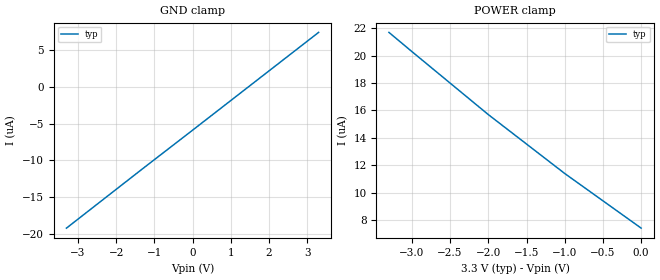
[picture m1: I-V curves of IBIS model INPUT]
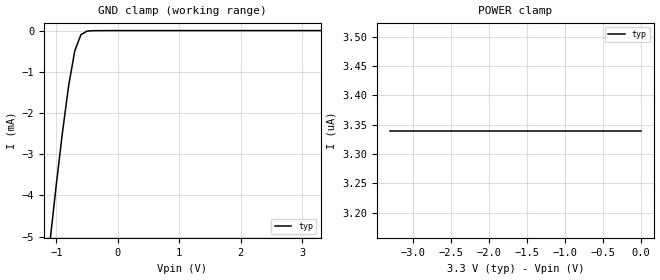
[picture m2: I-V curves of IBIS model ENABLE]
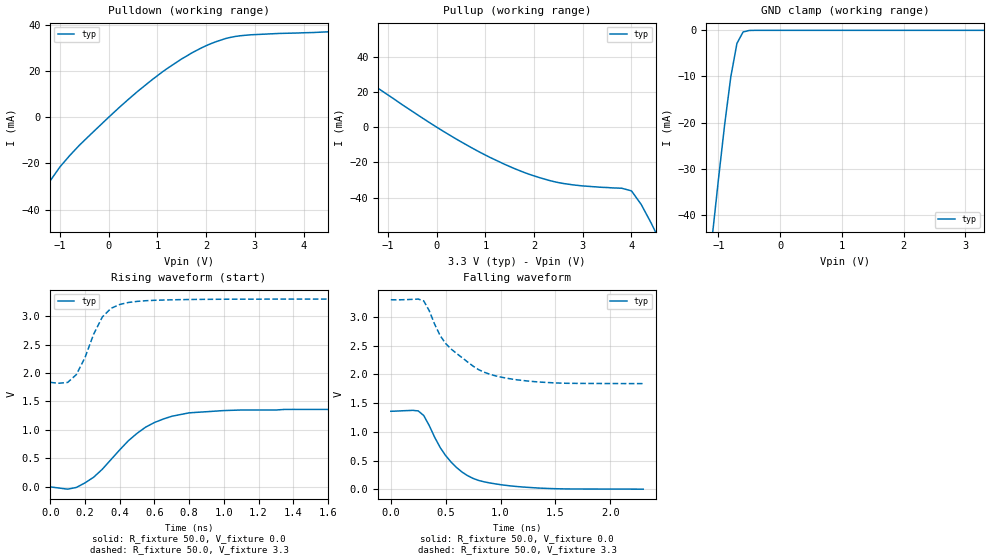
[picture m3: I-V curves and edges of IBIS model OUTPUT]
|   Texas Instruments Incorporated
|   Data Transmissions Products
|   IBIS Model for SN55LVDS33
|   16W CPK Package
[IBIS Ver]   3.2
[Comment char]   |_char
[File name]   lvds33w.ibs
[File Rev]   1.0
[Date]   26Mar01
[Source]   File originated at Texas Instruments Incorporated.
   Data Transmission Products Group. All data based on
   Bench Measurements.
[Notes]
   This file was modified on 4/14/2014 14:11 by the Mentor Graphics
   IBISVTC program, to remove initial non-switching delay(s) from one
   or more models V-t tables. Modified models:
   OUTPUT
   Original V-t tables have been left in the affected models, but commented out.
[Disclaimer]
(C) Copyright Texas Instruments Incorporated 2001
   All rights reserved
  Texas Instruments Incorporated hereby grants the user of this IBIS
model a non-exclusive, nontransferable license to use this IBIS model
under the following terms.  Before using this IBIS model, the user
should read this license.  If the user does not accept these terms,
the IBIS model should be returned to Texas Instruments within 30 days.
  The user is granted this license only to use the IBIS model and
is not granted rights to sell, load, rent, lease or license the IBIS
model in whole or in part, or in modified form to anyone other than
user.  User may modify the IBIS model to suit its specific applications
but rights to derivative works and such modifications shall belong to
Texas Instruments.
  This IBIS model is provided on an "AS IS" basis and Texas Instruments
makes absolutely no warranty with respect to the information contained
herein.  TEXAS INSTRUMENTS DISCLAIMS AND CUSTOMER WAIVES ALL WARRANTIES,
EXPRESS OR IMPLIED, INCLUDING WARRANTIES OF MERCHANTABILITY OR FITNESS
FOR A PARTICULAR PURPOSE. The entire risk as to quality and performance
is with the Customer. ACCORDINGLY, IN NO EVENT SHALL THE COMPANY BE LIABLE
FOR ANY DAMAGES, WHETHER IN CONTRACT OR TORT,INCLUDING ANY LOST PROFITS
OR OTHER INCIDENTAL, CONSEQUENTIAL, EXEMPLARY, OR PUNITIVE DAMAGES ARISING
OUT OF THE USE OR APPLICATION OF THE IBIS model provided in this package.
Further, Texas Instruments reserves the right to discontinue or make changes
without notice to any product herein to improve reliability, function, or
design. Texas Instruments does not convey any license under patent rights
or any other intellectual property rights, including those of third parties.
Contact Texas Instruments at ATTN:DATA TRANSMISSIONS
[Copyright]   Copyright 2001, Texas Instruments, All Rights Reserved
[Component]   SN55LVDS33W
[Manufacturer]  Texas Instruments Incorporated
[Package]
|   typ   min   max
R_pkg   0.177   0.141   0.245
L_pkg   3.23e-9   2.617e-9   4.412e-9
C_pkg   1.228e-12   1.057e-12   1.531e-12
[Pin]   signal_name   model_name   R_pin   L_pin   C_pin
1   1B   INPUT   0.244   4.385e-9 1.524e-12
2   1A   INPUT   0.176   3.183e-9 1.235e-12
3   1Y   OUTPUT   0.142   2.637e-9 1.071e-12
4   G   ENABLE   0.144   2.645e-9 1.060e-12
5   2Y   OUTPUT   0.147   2.708e-9 1.081e-12
6   2A   INPUT   0.144   2.687e-9 1.092e-12
7   2B   INPUT   0.176   3.182e-9 1.236e-12
8   GND   GND   0.245   4.412e-9 1.531e-12
9   3B   INPUT   0.245   4.411e-9 1.531e-12
10   3A   INPUT   0.176   3.183e-9 1.235e-12
11   3Y   OUTPUT   0.141   2.617e-9 1.063e-12
12   /G   ENABLE   0.144   2.639e-9 1.057e-12
13   4Y   OUTPUT   0.150   2.772e-9 1.102e-12
14   4A   INPUT   0.141   2.617e-9 1.063e-12
15   4B   INPUT   0.176   3.182e-9 1.235e-12
16   VCC   POWER   0.245   4.411e-9 1.531e-12
[Diff_pin]   inv_pin   vdiff   tdelay_typ   tdelay_min   tdelay_max
| The 'xA' pin is Diff_pin and the 'xB' pin is the inv_pin
2   1   50mV   0 0 0   | Vth  +/-50mV
6   7   50mV   0 0 0
10   9   50mV   0 0 0
14   15   50mV   0 0 0
| Models and submodels in the file (3): INPUT (Input), ENABLE (Input), OUTPUT (3-state)
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|   Receiver Input  MODEL
[Model]   INPUT
Model_type   Input
|Signals   1A,1B,2A,2B,3A,3B,4A,4B
Vinh = 2.0
Vinl = 0.8
|   typ   min   max
C_comp   1.0pF   NA   NA
|   typ   min   max
[Temperature Range]   25.0   NA   NA
[Voltage range]   3.3V   3.0V   3.6V
[GND_clamp]
|   Voltage   I(typ)   I(min)   I(max)
-3.3V     -19.2uA    NA         NA
-1.3V     -11.1uA    NA         NA
0V        -5.89uA    NA         NA
1.3V      -651nA     NA         NA
3.3V      7.41uA     NA         NA
[Power_clamp]
| Note that the[POWER_clamp]voltage table is referenced to Vcc
| and is calculated using Vtable=Vcc - Vmeasured.
|   Voltage   I(typ)   I(min)   I(max)
-3.3V     21.7uA     NA         NA
-3V       20.3uA     NA         NA
-2V       15.7uA     NA         NA
-1V       11.4uA     NA         NA
0V        7.41uA     NA         NA
|   Receiver Enable  MODEL
[Model]   ENABLE
Model_type   Input
|Signals   G,/G
Vinh = 2.0
Vinl = 0.8
|   typ   min   max
C_comp   1.0pF   NA   NA
|   typ   min   max
[Temperature Range]   25.0   NA   NA
[Voltage range]   3.3V   3.0V   3.6V
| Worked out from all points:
|   GND clamp passes 1 mA (typ) near -0.76 V on its own axis
[GND_clamp]
|   Voltage   I(typ)   I(min)   I(max)
-3.3V     -43.1mA    NA         NA
-1.1V     -5.08mA    NA         NA
-1V       -3.73mA    NA         NA
-900mV    -2.47mA    NA         NA
-800mV    -1.34mA    NA         NA
-700mV    -493uA     NA         NA
-600mV    -98.5uA    NA         NA
-500mV    -13.3uA    NA         NA
3.3V      3.34pA     NA         NA
[Power_clamp]
| Note that the[POWER_clamp]voltage table is referenced to Vcc
| and is calculated using Vtable=Vcc - Vmeasured.
|   Voltage   I(typ)   I(min)   I(max)
-3.3V     3.34uA     NA         NA
-2.7V     3.34uA     NA         NA
-2V       3.34uA     NA         NA
-800mV    3.34uA     NA         NA
0V        3.34uA     NA         NA
|   Receiver Output  MODEL
[Model]   OUTPUT
Model_type   3-state
| Signals   1Y,2Y,3Y,4Y
Vmeas = 1.5V   |Reference voltage for timing measurements
Cref = 8pF   |Timing specification test load capacitance value
Vref = 0   |Timing specification test load voltage; GND
| variable   typ   min   max
C_comp   1.0pF   NA   NA
|   typ   min   max
[Temperature Range]   25.0   NA   NA
[Voltage range]   3.3V   3.0V   3.6V
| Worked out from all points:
|   slope of the pulldown table from 0 to 0.495 V, typ, clamps not added: 52.7 ohm
|   slope of the pullup table from 0 to 0.495 V, typ, clamps not added: 60.3 ohm
|   GND clamp passes 1 mA (typ) near -0.63 V on its own axis
|   rising waveform, R_fixture 50.0, V_fixture 0.0: 20-80 % time 287ps typ, NA min, NA max; typ from 0 V to 1.36 V
|   falling waveform, R_fixture 50.0, V_fixture 0.0: 20-80 % time 315ps typ, NA min, NA max; typ from 1.36 V to 0.004 V
|   rising waveform, R_fixture 50.0, V_fixture 3.3: 20-80 % time 131ps typ, NA min, NA max; typ from 1.84 V to 3.3 V
|   falling waveform, R_fixture 50.0, V_fixture 3.3: 20-80 % time 389ps typ, NA min, NA max; typ from 3.3 V to 1.84 V
[Pulldown]
|   Voltage   I(typ)   I(min)   I(max)
-3.3V     -150mA     NA         NA
-1.6V     -47.9mA    NA         NA
-1.2V     -27.5mA    NA         NA
-1V       -21.5mA    NA         NA
-600mV    -12.1mA    NA         NA
200mV     3.91mA     NA         NA
900mV     16.4mA     NA         NA
1.5V      25.3mA     NA         NA
2.1V      31.9mA     NA         NA
2.5V      34.6mA     NA         NA
2.9V      35.7mA     NA         NA
6.6V      39.1mA     NA         NA
[Pullup]
|   Voltage   I(typ)   I(min)   I(max)
| Note that the[Pullup]voltage table is referenced to Vcc
| and is calculated using Vtable=Vcc - Vmeasured.
-3.3V     61mA       NA         NA
-3.1V     57.2mA     NA         NA
-3V       55.4mA     NA         NA
100mV     -1.72mA    NA         NA
900mV     -14.4mA    NA         NA
1.6V      -23.5mA    NA         NA
2.5V      -31.4mA    NA         NA
4V        -36.1mA    NA         NA
4.2V      -43.8mA    NA         NA
4.4V      -54.1mA    NA         NA
4.6V      -65.3mA    NA         NA
6.6V      -187mA     NA         NA
| Output in High Impedance (off)
[GND_clamp]
|   Voltage   I(typ)   I(min)   I(max)
-3.3V     -347mA     NA         NA
-1.1V     -44.7mA    NA         NA
-1V       -32.3mA    NA         NA
-900mV    -20.5mA    NA         NA
-800mV    -10.1mA    NA         NA
-700mV    -2.82mA    NA         NA
-600mV    -350uA     NA         NA
-500mV    -29.4uA    NA         NA
-400mV    -1.91uA    NA         NA
3.3V      426pA      NA         NA
[POWER_clamp]
|   Voltage   I(typ)   I(min)   I(max)
| Note that the [POWER_clamp] voltage table is referenced to Vcc
| and is calculated using Vtable = Vcc - Vmeasured.
| Outputs in Tri-state.
-3.3V     0A         NA         NA
0V        0A         NA         NA
[Ramp]
|   typ   min   max
dV/dt_r   0.815V/389ps   NA   NA
dV/dt_f   0.880V/285ps   NA   NA
R_load = 50
[Rising Waveform]
R_fixture = 50.0
V_fixture = 0.0
C_fixture = 0p
L_fixture = 0n
|   V(typ)   V(min)   V(max)
|   7.00E-09   0.00   NA   NA
|   7.85E-09   0.00   NA   NA
|   7.90E-09   -0.02   NA   NA
|   7.95E-09   -0.04   NA   NA
|   8.00E-09   -0.01   NA   NA
|   8.05E-09   0.07   NA   NA
|   8.10E-09   0.17   NA   NA
|   8.15E-09   0.31   NA   NA
|   8.20E-09   0.48   NA   NA
|   8.25E-09   0.65   NA   NA
|   8.30E-09   0.81   NA   NA
|   8.35E-09   0.94   NA   NA
|   8.40E-09   1.05   NA   NA
|   8.45E-09   1.13   NA   NA
|   8.50E-09   1.19   NA   NA
|   8.55E-09   1.24   NA   NA
|   8.60E-09   1.27   NA   NA
|   8.65E-09   1.30   NA   NA
|   8.70E-09   1.31   NA   NA
|   8.75E-09   1.32   NA   NA
|   8.80E-09   1.33   NA   NA
|   8.85E-09   1.34   NA   NA
|   8.95E-09   1.35   NA   NA
|   9.15E-09   1.35   NA   NA
|   9.20E-09   1.36   NA   NA
|   1.00E-08   1.36   NA   NA
0s        0V         NA         NA
100ps     -40mV      NA         NA
200ps     70mV       NA         NA
300ps     310mV      NA         NA
500ps     940mV      NA         NA
600ps     1.13V      NA         NA
700ps     1.24V      NA         NA
800ps     1.3V       NA         NA
1.1ns     1.35V      NA         NA
2.15ns    1.36V      NA         NA
[Falling Waveform]
R_fixture = 50.0
V_fixture = 0.0
C_fixture = 0p
L_fixture = 0n
|   V(typ)   V(min)   V(max)
|   1.200E-08   1.359   NA   NA
|   1.240E-08   1.358   NA   NA
|   1.270E-08   1.360   NA   NA
|   1.275E-08   1.362   NA   NA
|   1.280E-08   1.367   NA   NA
|   1.285E-08   1.371   NA   NA
|   1.290E-08   1.375   NA   NA
|   1.295E-08   1.365   NA   NA
|   1.300E-08   1.285   NA   NA
|   1.305E-08   1.111   NA   NA
|   1.310E-08   0.905   NA   NA
|   1.315E-08   0.728   NA   NA
|   1.320E-08   0.587   NA   NA
|   1.325E-08   0.474   NA   NA
|   1.330E-08   0.379   NA   NA
|   1.335E-08   0.300   NA   NA
|   1.340E-08   0.239   NA   NA
|   1.345E-08   0.191   NA   NA
|   1.350E-08   0.156   NA   NA
|   1.355E-08   0.132   NA   NA
|   1.360E-08   0.113   NA   NA
|   1.365E-08   0.097   NA   NA
|   1.370E-08   0.082   NA   NA
|   1.375E-08   0.070   NA   NA
|   1.380E-08   0.059   NA   NA
|   1.385E-08   0.050   NA   NA
|   1.390E-08   0.042   NA   NA
|   1.395E-08   0.035   NA   NA
|   1.400E-08   0.029   NA   NA
|   1.405E-08   0.023   NA   NA
|   1.410E-08   0.019   NA   NA
|   1.415E-08   0.015   NA   NA
|   1.420E-08   0.012   NA   NA
|   1.425E-08   0.010   NA   NA
|   1.430E-08   0.008   NA   NA
|   1.440E-08   0.007   NA   NA
|   1.460E-08   0.006   NA   NA
|   1.485E-08   0.005   NA   NA
|   1.500E-08   0.004   NA   NA
0s        1.359V     NA         NA
250ps     1.365V     NA         NA
300ps     1.285V     NA         NA
450ps     728mV      NA         NA
550ps     474mV      NA         NA
650ps     300mV      NA         NA
800ps     156mV      NA         NA
1ns       82mV       NA         NA
1.35ns    23mV       NA         NA
2.3ns     4mV        NA         NA
[Rising Waveform]
R_fixture = 50.0
V_fixture = 3.3
C_fixture = 0p
L_fixture = 0n
|   V(typ)   V(min)   V(max)
|   7.00E-09   1.836   NA   NA
|   7.60E-09   1.835   NA   NA
|   7.65E-09   1.833   NA   NA
|   7.70E-09   1.830   NA   NA
|   7.75E-09   1.826   NA   NA
|   7.80E-09   1.824   NA   NA
|   7.85E-09   1.826   NA   NA
|   7.90E-09   1.820   NA   NA
|   7.95E-09   1.834   NA   NA
|   8.00E-09   1.971   NA   NA
|   8.05E-09   2.270   NA   NA
|   8.10E-09   2.682   NA   NA
|   8.15E-09   2.984   NA   NA
|   8.20E-09   3.135   NA   NA
|   8.25E-09   3.203   NA   NA
|   8.30E-09   3.238   NA   NA
|   8.35E-09   3.257   NA   NA
|   8.40E-09   3.269   NA   NA
|   8.45E-09   3.276   NA   NA
|   8.50E-09   3.281   NA   NA
|   8.55E-09   3.285   NA   NA
|   8.60E-09   3.288   NA   NA
|   8.65E-09   3.290   NA   NA
|   8.70E-09   3.292   NA   NA
|   8.75E-09   3.293   NA   NA
|   8.80E-09   3.294   NA   NA
|   8.85E-09   3.295   NA   NA
|   8.95E-09   3.296   NA   NA
|   9.05E-09   3.296   NA   NA
|   9.10E-09   3.297   NA   NA
|   9.35E-09   3.297   NA   NA
|   9.40E-09   3.298   NA   NA
|   1.00E-08   3.298   NA   NA
0s        1.836V     NA         NA
100ps     1.834V     NA         NA
150ps     1.971V     NA         NA
200ps     2.27V      NA         NA
250ps     2.682V     NA         NA
300ps     2.984V     NA         NA
350ps     3.135V     NA         NA
450ps     3.238V     NA         NA
850ps     3.292V     NA         NA
2.15ns    3.298V     NA         NA
[Falling Waveform]
R_fixture = 50.0
V_fixture = 3.3
C_fixture = 0p
L_fixture = 0n
|   V(typ)   V(min)   V(max)
|   1.200E-08   3.299   NA   NA
|   1.205E-08   3.300   NA   NA
|   1.260E-08   3.299   NA   NA
|   1.265E-08   3.298   NA   NA
|   1.275E-08   3.298   NA   NA
|   1.280E-08   3.299   NA   NA
|   1.285E-08   3.302   NA   NA
|   1.290E-08   3.306   NA   NA
|   1.295E-08   3.311   NA   NA
|   1.300E-08   3.279   NA   NA
|   1.305E-08   3.109   NA   NA
|   1.310E-08   2.871   NA   NA
|   1.315E-08   2.674   NA   NA
|   1.320E-08   2.537   NA   NA
|   1.325E-08   2.441   NA   NA
|   1.330E-08   2.364   NA   NA
|   1.335E-08   2.291   NA   NA
|   1.340E-08   2.216   NA   NA
|   1.345E-08   2.144   NA   NA
|   1.350E-08   2.083   NA   NA
|   1.355E-08   2.039   NA   NA
|   1.360E-08   2.005   NA   NA
|   1.365E-08   1.977   NA   NA
|   1.370E-08   1.955   NA   NA
|   1.375E-08   1.936   NA   NA
|   1.380E-08   1.920   NA   NA
|   1.385E-08   1.906   NA   NA
|   1.390E-08   1.895   NA   NA
|   1.395E-08   1.885   NA   NA
|   1.400E-08   1.876   NA   NA
|   1.405E-08   1.868   NA   NA
|   1.410E-08   1.862   NA   NA
|   1.415E-08   1.857   NA   NA
|   1.420E-08   1.852   NA   NA
|   1.425E-08   1.849   NA   NA
|   1.430E-08   1.846   NA   NA
|   1.440E-08   1.844   NA   NA
|   1.450E-08   1.843   NA   NA
|   1.465E-08   1.842   NA   NA
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0s        3.299V     NA         NA
250ps     3.311V     NA         NA
300ps     3.279V     NA         NA
350ps     3.109V     NA         NA
450ps     2.674V     NA         NA
500ps     2.537V     NA         NA
750ps     2.144V     NA         NA
900ps     2.005V     NA         NA
1.4ns     1.862V     NA         NA
2.3ns     1.84V      NA         NA
